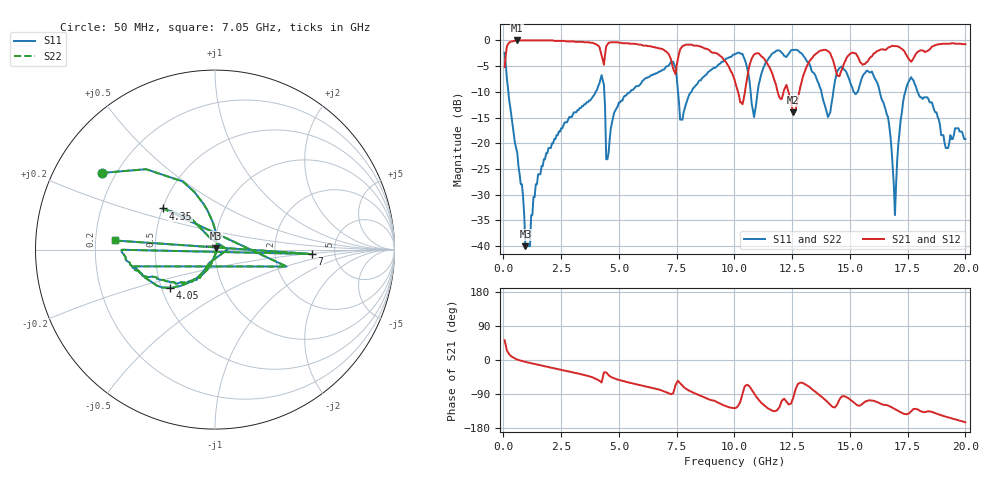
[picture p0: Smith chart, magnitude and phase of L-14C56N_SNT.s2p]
#	mhz	s	ma	r	50
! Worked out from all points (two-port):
!   400 points, 50 MHz to 20 GHz, reference 50 ohm
!   highest |S21| = 0.00 dB at 600 MHz (marker M1); lowest = -14.0 dB at 12.55 GHz (marker M2)
!   |S21| within 3 dB of the highest: 96.87 MHz to 4.258 GHz (4.161 GHz wide, 191 % of centre); 4.393 GHz to 7.19 GHz (2.797 GHz wide, 48.3 % of centre)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
!   lowest |S11| = -40.0 dB at 950 MHz (marker M3), VSWR 1.02, Z = 50.6 + j0.803 ohm
!   |S11| at or under -10 dB: 213.5 MHz to 3.991 GHz (3.777 GHz wide, 180 % of centre); 4.365 GHz to 5.481 GHz (1.116 GHz wide, 22.7 % of centre); 17.93 GHz to end of sweep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
!   |S22| runs from -40.0 to -1.8 dB; largest |S21 - S12| = 0
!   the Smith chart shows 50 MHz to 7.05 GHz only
!   S11 on the Smith chart (normalised r, x): 50 MHz: 0.15, +0.30; 4.05 GHz: 0.55, -0.26; 4.35 GHz: 0.50, +0.27; 7 GHz: 3.33, -0.23; 7.05 GHz: 0.28, +0.04
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50  0.76 145.8  0.55 52.1  0.55 52.1  0.76 145.8
600  0.08 83.1  1 1.2  1 1.2  0.08 83.1
950  0.01 52.5  1 -5.0  1 -5.0  0.01 52.5
3400  0.23 -127.7  0.97 -38.2  0.97 -38.2  0.23 -127.7
4050  0.33 -140.0  0.91 -50.8  0.91 -50.8  0.33 -140.0
4250  0.46 -168.3  0.72 -59.3  0.72 -59.3  0.46 -168.3
4300  0.41 -13.3  0.65 -45.9  0.65 -45.9  0.41 -13.3
4350  0.37 141.7  0.58 -32.5  0.58 -32.5  0.37 141.7
4500  0.07 -0.2  0.91 -36.3  0.91 -36.3  0.07 -0.2
6700  0.49 -172.2  0.84 -77.5  0.84 -77.5  0.49 -172.2
6950  0.52 -179.9  0.81 -82.3  0.81 -82.3  0.52 -179.9
7000  0.54 -2.6  0.79 -83.7  0.79 -83.7  0.54 -2.6
7050  0.56 174.8  0.78 -85.1  0.78 -85.1  0.56 174.8
7750  0.17 163.7  0.88 -68.4  0.88 -68.4  0.17 163.7
10050  0.74 125.4  0.38 -126.9  0.38 -126.9  0.74 125.4
10850  0.18 118.5  0.73 -87.8  0.73 -87.8  0.18 118.5
12550  0.81 87.2  0.2 -98.8  0.2 -98.8  0.81 87.2
13350  0.5 44.2  0.67 -76.7  0.67 -76.7  0.5 44.2
16700  0.15 -21.4  0.86 -121.5  0.86 -121.5  0.15 -21.4
16950  0.02 25.8  0.88 -129.7  0.88 -129.7  0.02 25.8
17650  0.44 55.1  0.62 -135.5  0.62 -135.5  0.44 55.1
20000  0.11 -87.1  0.92 -164.5  0.92 -164.5  0.11 -87.1
